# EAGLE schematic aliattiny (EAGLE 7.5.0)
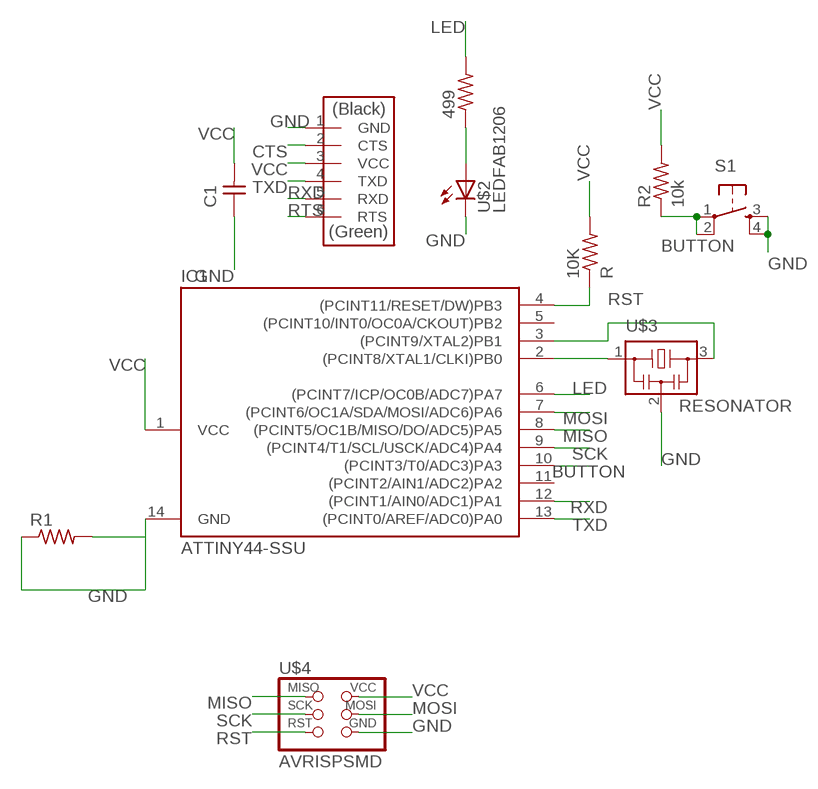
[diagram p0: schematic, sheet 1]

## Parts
10K  R  RES-US1206FAB  [R1206FAB]
499  RES-US1206FAB  [R1206FAB]
C1  CAP-UNPOLARIZEDFAB  [C1206FAB]
IC1  ATTINY44-SSU  [SOIC14]
R1  RES-US1206FAB  [R1206FAB]
R2  10k  RES-US1206FAB  [R1206FAB]
S1  6MM_SWITCH6MM_SWITCH  [6MM_SWITCH]
U$1  FTDI-SMD-HEADER  [1X06SMD]
U$2  LEDFAB1206  [LED1206FAB]
U$3  RESONATOR  [EFOBM]
U$4  AVRISPSMD  [2X03SMD]

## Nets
BUTTON: IC1.10((PCINT3/T0/ADC3)PA3) R2.1 S1.1(P) S1.2(P1)
CTS: U$1.2(CTS)
GND: C1.1 IC1.14(GND) R1.1 R1.2 S1.3(S) S1.4(S1) U$1.1(GND) U$2.2(C) U$3.2 U$4.6(GND)
LED: 499.2 IC1.6((PCINT7/ICP/OC0B/ADC7)PA7)
MISO: IC1.8((PCINT5/OC1B/MISO/DO/ADC5)PA5) U$4.1(MISO)
MOSI: IC1.7((PCINT6/OC1A/SDA/MOSI/ADC6)PA6) U$4.4(MOSI)
N$4: IC1.2((PCINT8/XTAL1/CLKI)PB0) U$3.1
N$5: IC1.3((PCINT9/XTAL2)PB1) U$3.3
N$6: 499.1 U$2.1(A)
RST: 10K.1 IC1.4((PCINT11/RESET/DW)PB3) U$4.5(RST)
RTS: U$1.6(RTS)
RXD: IC1.12((PCINT1/AIN0/ADC1)PA1) U$1.5(RXD)
SCK: IC1.9((PCINT4/T1/SCL/USCK/ADC4)PA4) U$4.3(SCK)
TXD: IC1.13((PCINT0/AREF/ADC0)PA0) U$1.4(TXD)
VCC: 10K.2 C1.2 IC1.1(VCC) R2.2 U$1.3(VCC) U$4.2(VCC)
Unconnected: IC1.5((PCINT10/INT0/OC0A/CKOUT)PB2) IC1.11((PCINT2/AIN1/ADC2)PA2)

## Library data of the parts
10K 499 R1 R2 = fab:RES-US: Resistor (US Symbol)
C1 = fab:CAP-UNPOLARIZED
IC1 = fab:ATTINY44
S1 = fab:6MM_SWITCH: OMRON SWITCH
U$1 = fab:FTDI-SMD-HEADER
U$2 = fab:LED: LED
U$3 = fab:RESONATOR
U$4 = fab:AVRISP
